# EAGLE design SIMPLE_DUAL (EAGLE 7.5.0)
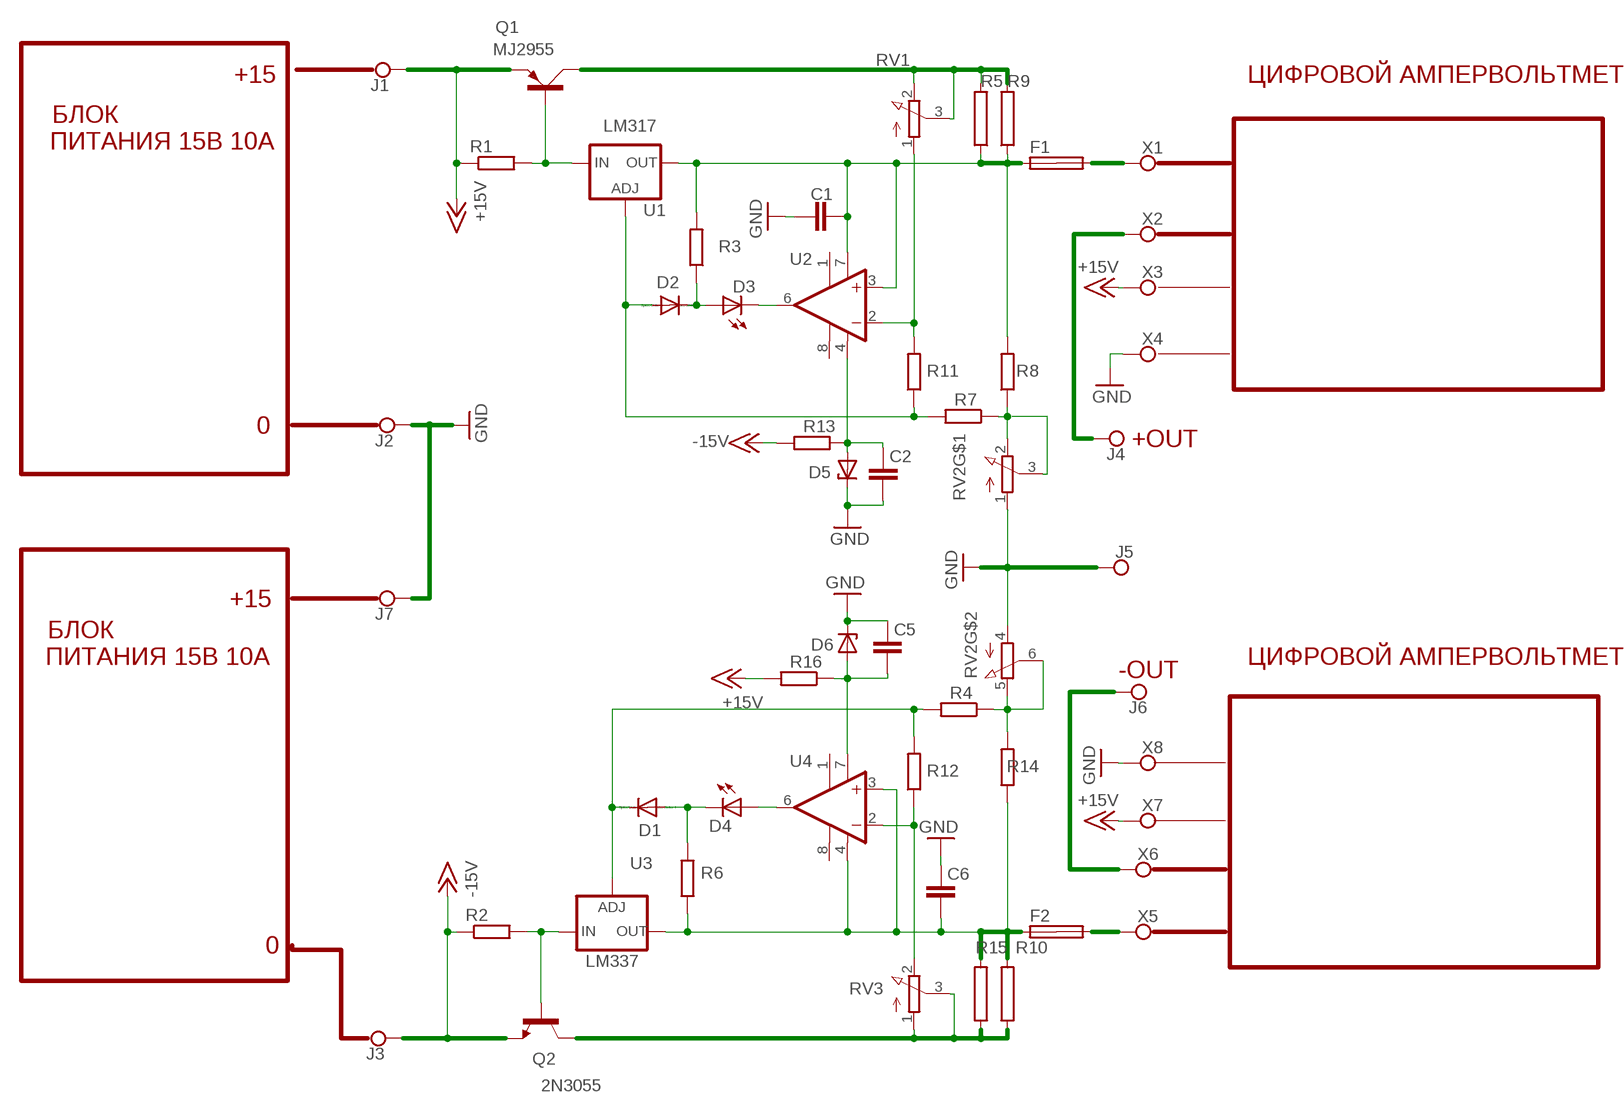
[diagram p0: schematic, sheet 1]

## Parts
C1  C-EUC1206  [C1206]
C2  C-EUC1206  [C1206]
C5  C-EUC1206  [C1206]
C6  C-EUC1206  [C1206]
D1  1N4148DO35-10  [DO35-10]
D2  1N4148DO35-10  [DO35-10]
D3  LED5MM  [LED5MM]
D4  LED5MM  [LED5MM]
D5  BZX85  [DO41Z10]
D6  BZX85  [DO41Z10]
F1  SHK20L  [SHK20L]
F2  SHK20L  [SHK20L]
J1  TPPAD1-20  [P1-20]
J2  TPPAD1-20  [P1-20]
J3  TPPAD1-20  [P1-20]
J4  TPPAD1-20  [P1-20]
J5  TPPAD1-20  [P1-20]
J6  TPPAD1-20  [P1-20]
J7  TPPAD1-20  [P1-20]
Q1  MJ2955  [TO3A]
Q2  2N3055  [TO3]
R1  R-EU_0207/10  [0207/10]
R2  R-EU_0207/10  [0207/10]
R3  R-EU_0207/10  [0207/10]
R4  R-EU_0207/10  [0207/10]
R5  RKH208-8  [KH208-8]
R6  R-EU_0207/10  [0207/10]
R7  R-EU_0207/10  [0207/10]
R8  R-EU_0207/10  [0207/10]
R9  RKH208-8  [KH208-8]
R10  RKH208-8  [KH208-8]
R11  R-EU_0207/10  [0207/10]
R12  R-EU_0207/10  [0207/10]
R13  R-EU_0207/10  [0207/10]
R14  R-EU_0207/10  [0207/10]
R15  RKH208-8  [KH208-8]
R16  R-EU_0207/10  [0207/10]
RV1  PTV111  [PTV111]
RV2  PTV112  [PTV112]
RV3  PTV111  [PTV111]
U1  LM317-TO3  [TO3-K02]
U2  OPA177P  [DIL08]
U3  LM337-TO3  [TO3-K02]
U4  OPA177P  [DIL08]
X1  TPPAD1-20  [P1-20]
X2  TPPAD1-20  [P1-20]
X3  TPPAD1-20  [P1-20]
X4  TPPAD1-20  [P1-20]
X5  TPPAD1-20  [P1-20]
X6  TPPAD1-20  [P1-20]
X7  TPPAD1-20  [P1-20]
X8  TPPAD1-20  [P1-20]

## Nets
+15V: J1.TP Q1.E R1.1 R16.2 X3.TP X7.TP
-15V: J3.TP Q2.E R2.1 R13.2
GND: C1.1 C2.1 C5.2 C6.2 D5.C D6.C J2.TP J5.TP J7.TP RV2.1(A) RV2.4(A) X4.TP X8.TP
N$1: Q1.B R1.2 U1.1(IN)
N$2: F1.2A X1.TP
N$3: Q2.B R2.2 U3.3(IN)
N$4: J4.TP X2.TP
N$5: Q1.C Q1.C1(C) R5.2 R9.2 RV1.2(E) RV1.3(S)
N$6: R11.2 RV1.1(A) U2.2(-IN)
N$7: D2.A R7.2 R11.1 U1.2(ADJ)
N$8: C1.2 F1.1A R3.2 R5.1 R8.2 R9.1 U1.3(OUT) U2.3(+IN) U2.7(V+)
N$9: R7.1 R8.1 RV2.2(E)
N$10: RV2.3(S)
N$11: D2.C D3.A R3.1
N$12: D3.K(C) U2.6(OUT)
N$13: C2.2 D5.A R13.1 U2.4(V-)
N$14: Q2.C Q2.C/(C) R10.1 R15.1 RV3.1(A) RV3.3(S)
N$16: D1.C R4.2 R12.2 U3.2(ADJ)
N$17: R4.1 R14.2 RV2.5(E) RV2.6(S)
N$18: R12.1 RV3.2(E) U4.2(-IN)
N$19: D4.A U4.6(OUT)
N$20: D1.A D4.K(C) R6.2
N$21: C5.1 D6.A R16.1 U4.7(V+)
N$22: F2.2A X5.TP
N$23: C6.1 F2.1A R6.1 R10.2 R14.1 R15.2 U3.1(OUT) U4.3(+IN) U4.4(V-)
N$24: J6.TP X6.TP
Unconnected: F1.1B F1.2B F2.1B F2.2B U2.1(TRIM1) U2.8(TRIM2) U4.1(TRIM1) U4.8(TRIM2)

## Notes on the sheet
- +15 | ЦИФРОВОЙ АМПЕРВОЛЬТМЕТР
- БЛОК
- LM317
- ПИТАНИЯ 15В 10А
- 0
- +OUT
- +15
- БЛОК
- ПИТАНИЯ 15В 10А | ЦИФРОВОЙ АМПЕРВОЛЬТМЕТР
- -OUT
- 0
- LM337

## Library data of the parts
C1 C2 C5 C6 = rcl:C-EU: CAPACITOR, European symbol
D1 D2 = diode:1N4148: DIODE
D3 D4 = led:LED: LED
D5 D6 = diode:BZX85: Z DIODE
F1 F2 = fuse:SHK20L: FUSE HOLDER 5 x 20 mm, SH contact, SHH1 Schukat, E1073 Buerklin; OC_FARNELL: unknown; OC_NEWARK: unknown
J1-J7 X1-X8 = testpad:TP: Test pad
Q1 = transistor-power:MJ2955: PNP TRANSISTOR
Q2 = transistor:2N3055: NPN TRANSISTOR
R1-R4 R6-R8 R11-R14 R16 = rcl:R-EU_: RESISTOR, European symbol
R5 R9 R10 R15 = resistor-power:R: Power Resitor; OC_FARNELL: unknown; OC_NEWARK: unknown
RV1 RV3 = pot:PTV111
RV2 = pot:PTV112
U1 = v-reg:LM317-TO3: VOLTAGE REGULATOR
U2 U4 = burr-brown:OPA177: Precision Operational Amplifier; MPN: OPA177GPG4; OC_FARNELL: 1219410; OC_NEWARK: 05M0933
U3 = v-reg:LM337-TO3: VOLTAGE REGULATOR

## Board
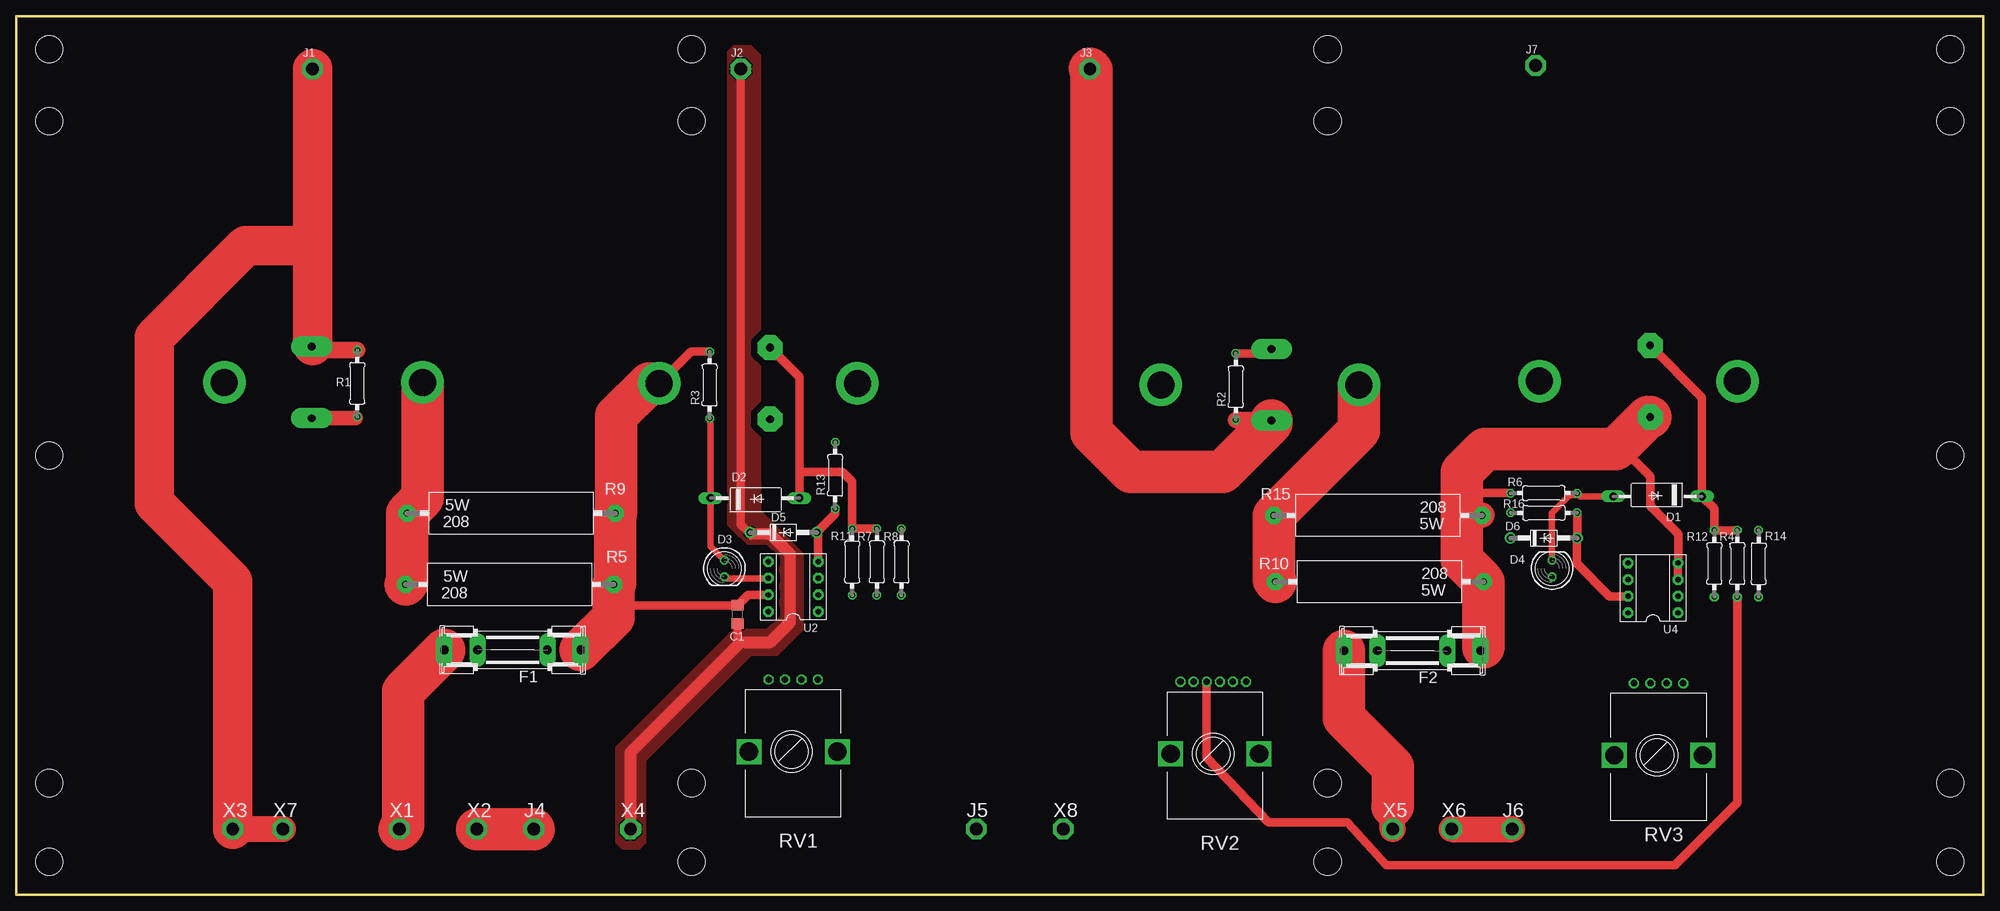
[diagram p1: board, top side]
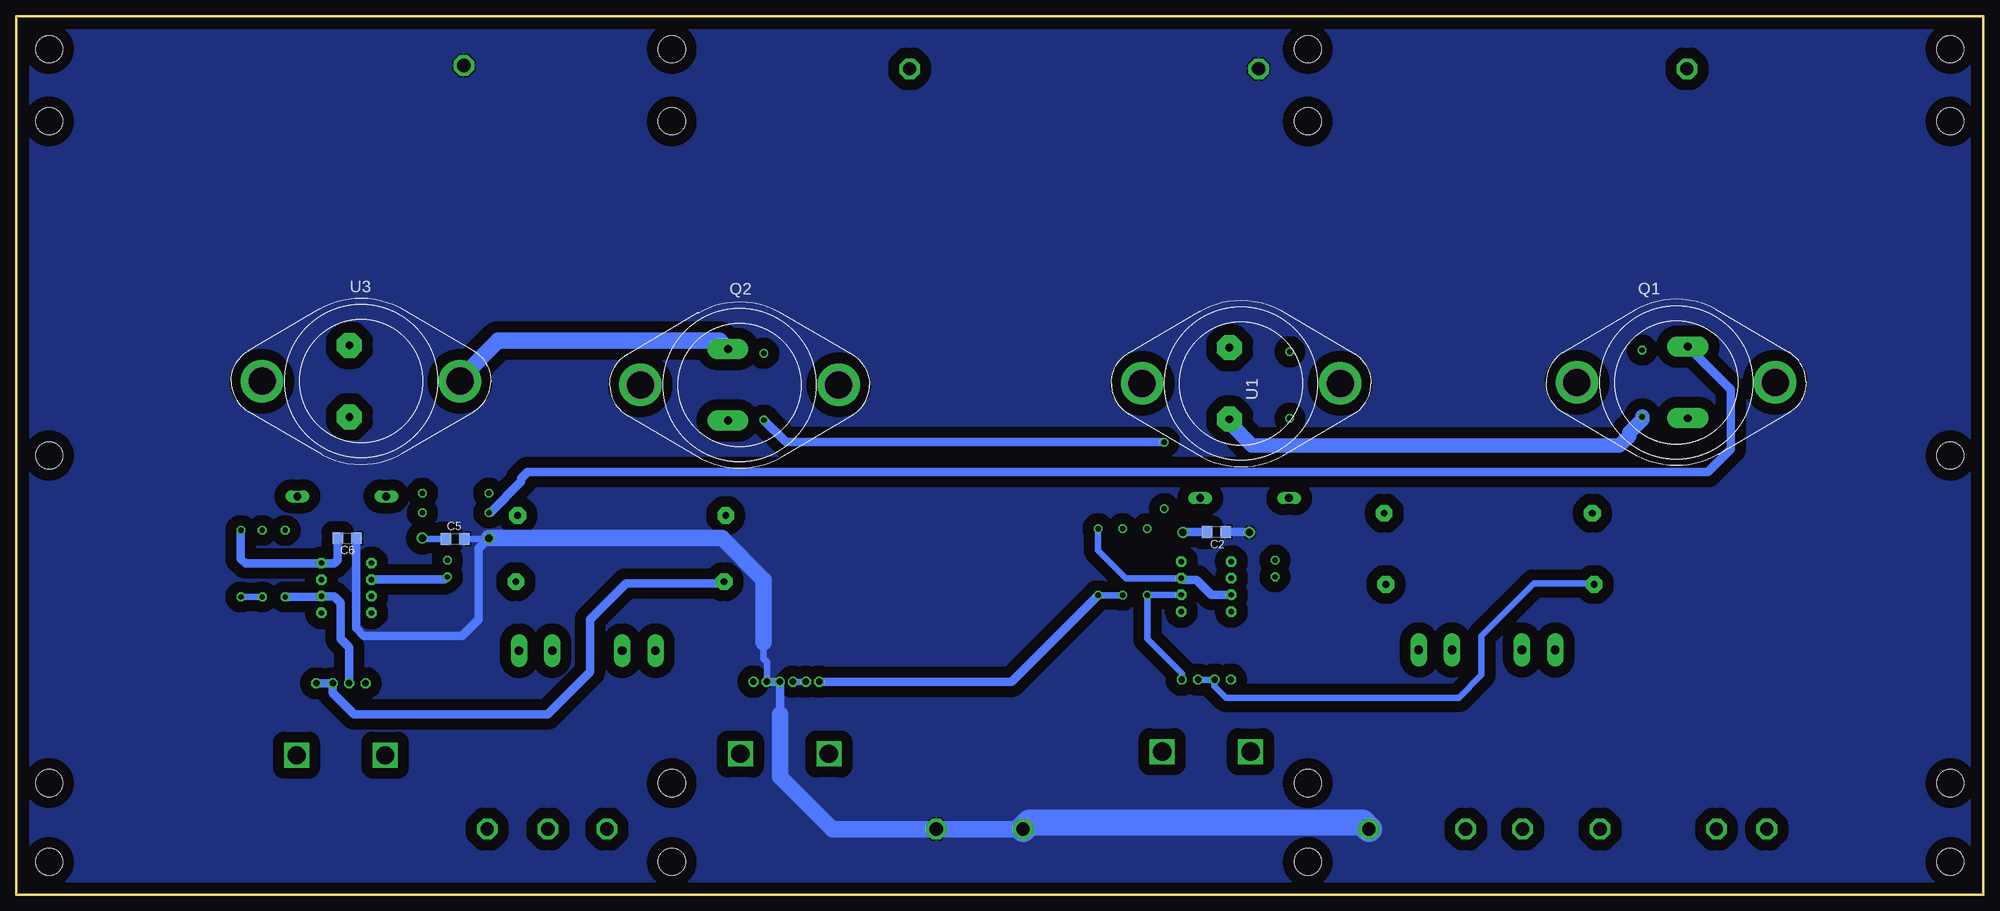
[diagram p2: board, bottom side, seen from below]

Size 300 x 134 mm. Coordinates in mm from the lower left corner, seen from the top.
Outline: 0,0 300,0 300,134 0,134 0,0
Copper layers (1*16): Top 0.035mm / dielectric 1.5mm / Bottom 0.035mm
Design rules "default": minimum track width 10mil, minimum drill 24mil, track to track 8mil, track to pad 8mil, pad to pad 8mil, via to via 8mil, smd to smd 8mil, copper to edge 40mil, drill to drill 8mil, minimum pad ring 10mil, minimum via ring 8mil, stop-mask expansion 4mil, vias tented up to drill 0mil, thermal gap 10mil
Holes 4.2 mm at 5,129 295,129 103,129 200,129 5,5 5,67 103,5 200,5 295,5 295,67 5,118 103,118 200,118 295,118 5,17 103,17 200,17 295,17

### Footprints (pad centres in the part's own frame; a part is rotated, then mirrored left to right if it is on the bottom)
C1206 = smd 1.6 x 1.8: 1 -1.4,0; 2 1.4,0
DO35-10 = drill 1.2 long: A 8.18,0; C -5.38,0
LED5MM = drill 0.813 octagon: A -1.27,0; K 1.27,0
DO41Z10 = drill 1.118: A 5.08,0; C -5.08,0
SHK20L = drill 1.321 pad 2.54 long: 1A -10.414,0; 1B -5.334,0; 2A 10.414,0; 2B 5.334,0
P1-20 = drill 2.007 pad 3.15 octagon: TP 0,0
TO3A = drill 1.194 pad 3.15 long: B -1.778,5.461; E -1.778,-5.461 | drill 4.115 pad 6.477: C 15.113,0; C1 -15.113,0
TO3 = drill 1.194 pad 3.15 long: B -1.778,5.461; E -1.778,-5.461 | drill 4.115 pad 6.477: C 15.113,0; C/ -15.113,0
0207/10 = drill 0.813 octagon: 1 -5.08,0; 2 5.08,0
KH208-8 = drill 1.016 pad 2.54 octagon: 1 -15.875,0; 2 15.875,0
PTV111 = drill 1 octagon: 1 3,-11; 2 8,-11; 3 5.5,-11; 4 10.5,-11 | drill 2.8 square: P$1 0,0; P$2 13.5,0
PTV112 = drill 1 octagon: 1 4,-11; 2 12,-11; 3 2,-11; 4 6,-11; 5 10,-11; 6 8,-11 | drill 2.8 square: P$1 0,0; P$2 13.5,0
TO3-K02 = drill 1.194 pad 3.81 octagon: 1 -1.778,-5.461; 2 -1.778,5.461 | drill 4.115 pad 6.477: 3 15.113,0; 3@ -15.113,0
DIL08 = drill 0.813 pad 1.6 octagon: 1 -3.81,-3.81; 2 -1.27,-3.81; 3 1.27,-3.81; 4 3.81,-3.81; 5 3.81,3.81; 6 1.27,3.81; 7 -1.27,3.81; 8 -3.81,3.81

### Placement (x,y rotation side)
C1  110,42.75 90 top
C2  116.96,55.31 180 bottom
C5  233.07,54.28 0 bottom
C6  249.57,54.37 0 bottom
D1  251.75,60.75 180 top
D2  111.25,60.5 0 top
D3  108,49.75 270 top
D4  234.25,49.75 90 top
D5  117,55.25 0 top
D6  232.99,54.38 0 top
F1  75.68,37.33 180 top
F2  212.93,37.22 180 top
J1  45.18,126 0 top
J2  110.5,126 0 top
J3  163.75,126 0 top
J4  78.93,10 0 top
J5  146.43,10 0 top
J6  228.18,10 0 top
J7  231.75,126.5 0 top
Q1  46.82,78.14 180 bottom
Q2  189.68,77.78 0 bottom
R1  52,78 270 top
R2  186,77.5 90 top
R3  105.75,77.75 90 top
R4  262.5,50.5 90 top
R5  75.22,47.32 180 top
R6  233,61.25 0 top
R7  131.25,50.75 90 top
R8  135,50.75 90 top
R9  75.47,58.19 180 top
R10  207.93,47.74 0 top
R11  127.5,50.75 270 top
R12  259,50.5 90 top
R13  124.9,63.96 90 top
R14  265.75,50.5 270 top
R15  207.68,57.86 0 top
R16  233,58.25 180 top
RV1  125.24,21.8 180 top
RV2  189.56,21.47 180 top
RV3  257.25,21.25 180 top
U1  113.18,77.99 0 bottom
U2  118.5,47 90 top
U3  247.43,78.34 0 bottom
U4  249.65,46.79 90 top
X1  58.43,10 0 top
X2  70.25,10 0 top
X3  33,10 0 top
X4  93.68,10 0 top
X5  209.93,10 0 top
X6  218.93,10 0 top
X7  40.68,10 0 top
X8  159.68,10 0 top

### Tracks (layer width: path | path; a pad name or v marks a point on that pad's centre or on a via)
+15V
  Top 1.016: 45.56,83.08 Q1.E
  Top 2.54: R1.1 45.56,83.08
  Top 4: 45.18,83.74 Q1.E | 44.93,99 45.18,98.75 | X7.TP X3.TP
  Top 6: J1.TP 45.18,98.75 45.18,83.74 | X3.TP 33,47.75 21,59.75 21,85 35,99 44.93,99
  Bottom 1.27: R16.2 227.75,58.25 223,63 223,63.5 222,64.5 42,64.5 38.5,68 38.5,77.06 Q1.E
-15V
  Top 2.54: R2.1 191.36,72.42 Q2.E
  Top 6.452: Q2.E 191.46,71.96 184,64.5 170,64.5 164,70.5 164,125.75 J3.TP
  Bottom 1.27: R13.2 182.62,69.04 R2.1
GND
  Top 1.27: C1.1 110,38.5 110.25,38.25 | D5.C 111.75,55.25 110.5,56.5 J2.TP
  Top 1.778: X4.TP 93.68,21.68 110.25,38.25 110.5,38.5 115,38.5 118,41.5 118,52 115,55 112.17,55 D5.C
  Bottom 1.016: 186,38.5 186,36 185.5,35.5 185.5,32.53 RV2.1 | C5.2 228.01,54.28 D6.C
  Bottom 1.27: C6.2 248.17,40.67 247,39.5 232,39.5 229.5,42 229.5,52.79 D6.C | C2.1 111.98,55.31 D5.C | 183.5,27.5 183.5,32.41 RV2.4 RV2.1
  Bottom 2.54: J5.TP X8.TP 175.5,10 183.5,18 183.5,27.5 | D6.C 192.38,54.38 186,48 186,38.5
  Bottom 4: J5.TP 146.43,10.07 145.5,11 94.68,11 X4.TP
  pour Bottom (isolate 1.676): 1,132.5 299,132.5 299,1 1,1
  pour Top (isolate 1.016): 109.5,129.5 112,129.5 113.5,128 113.5,58.5 120,52 120,40.5 116,36.5 112,36.5 96,20.5 96,8 95,7 92.5,7 91.5,8 91.5,22.5 109.5,40.5 114.5,40.5 116.5,42.5 116.5,51.5 114.5,53.5 111.5,53.5 109.5,55.5 108.5,56.5 108.5,128.5
N$1
  Top 1.27: 51.76,72.68 R1.2
  Top 2.184: Q1.B 51.76,72.68
  Bottom 2.184: R1.2 52,72.5 54,70.5 54,70 55.5,68.5 111.5,68.5 115,72 115,72.49 U1.1
N$2
  Top 6.452: F1.2A 65.27,37.27 59,31 59,10.57 X1.TP
N$3
  Top 1.27: R2.2 190.8,82.58 Q2.B
  Bottom 2.54: U3.3 232.32,78.68 226.5,84.5 192.72,84.5 Q2.B
N$4
  Top 6.452: X2.TP J4.TP
N$5
  Top 6.452: Q1.C 61.93,60.53 R9.2 59.59,47.57 R5.2
  Bottom 1.016: 59.16,47.5 68.5,47.5 76.5,39.5 76.5,33.5 80,30 115.5,30 117.24,31.74 RV1.2 RV1.3 | 59,47.5 59.16,47.5 | 59.16,47.5 R5.2
N$6
  Bottom 1.016: U2.2 127.44,45.73 R11.2 127.5,39 122.24,33.74 RV1.1
N$7
  Top 1.27: D2.A 119.43,64.5 | 119.43,64.5 119.43,78.98 U1.2 | R7.2 R11.1 127.5,63 126,64.5 119.43,64.5
N$8
  Top 1.27: U2.7 111.58,45.73 C1.2 91.75,44.15 91.75,43.74 91.5,43.5 90.5,43.5 90.5,42.5 91.09,42.5 | R3.2 102.91,82.83 U1.3
  Top 6.452: U1.3 96.49,77.99 91.5,73 91.5,58.34 R9.1 91.34,47.57 R5.1 91.09,42.5 91.09,42.33 F1.1A
  Bottom 1.016: U2.3 130.77,48.27 135,52.5 R8.2
  Bottom 1.27: U2.7 117.73,45.73 120,48 122.04,48 U2.3
N$9
  Bottom 1.016: R7.1 R8.1
  Bottom 1.27: RV2.2 148.2,32.47 R8.1
N$11
  Top 1.016: D3.A 105.87,53.15 D2.C 105.87,71.79 R3.1
N$12
  Top 1.016: U2.6 108.21,48.27 D3.K
N$13
  Top 1.27: U2.4 122.31,55.02 D5.A 124.9,58.07 R13.1
  Bottom 1.27: C2.2 122.02,55.31 D5.A
N$14
  Top 6.452: Q2.C/ 204.79,70.85 R15.1 191.81,47.99 R10.1
  Bottom 1.27: RV3.1 RV3.3 251.75,30.75 248.5,27.5 219,27.5 212.5,34 212.5,42 207,47.5 192.29,47.5 R10.1
N$16
  Top 1.27: R4.2 R12.2 259,58.88 D1.C 257.13,75.88 U3.2
N$17
  Top 1.27: RV2.6 181.56,20.94 191,11 203,11 209,4.5 253,4.5 262.5,14 R4.1
  Bottom 1.016: RV2.5 RV2.6 | R14.2 R4.1
N$18
  Bottom 1.27: R12.1 253.56,45.42 U4.2 253.44,45.5 251.5,45.5 250.5,44.5 250.5,39 249.25,37.75 RV3.2
N$19
  Bottom 1.27: U4.6 234.67,48.06 D4.A
N$20
  Top 1.016: D4.K 234.25,58.25 237,61 237.83,61 R6.2 238.58,60.75 D1.A
N$21
  Top 1.27: R16.1 D6.A 238,54.31 238,50.5 242.98,45.52 U4.7
  Bottom 1.016: C5.1 237.97,54.28 D6.A
N$22
  Top 4: X5.TP 209.93,13.5 209.93,17.43 210,17.5
  Top 6.452: F2.2A 202.52,29.52 202.5,29.5 202.5,27 210,19.5 210,13.57 209.93,13.5
N$23
  Top 1.27: U4.3 U4.4 253.5,50.64 253.5,55 249.21,59.29 249.21,63.79 244,69 244,68.5 243.5,68 | R6.1 222.25,61.25 222,61.5 222,59.5 221.5,59 222.41,59 R15.2
  Top 3.81: 223.56,47.99 223.56,48.45 221,51 221,58 223.41,58 R15.2
  Top 4: 223.81,37.68 F2.1A
  Top 6.452: 223.81,37.68 R10.2 223.56,47.99 220.5,51.05 220.5,64.5 224,68 243.5,68 244,68 248.88,72.88 U3.1
  Bottom 1.27: C6.1 250.97,51.03 251.5,50.5 253.36,50.5 U4.4 253.56,50.5 265,50.5 265.75,51.25 R14.1
N$24
  Top 4: X6.TP J6.TP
